(* Logix 5000 AddOnInstructionDefinition export Banner_Q90R_KD_Param_v4; software revision 33.00 *)

TYPE Banner_IOL_Port_v4 :   // UDT that has all of the data items necessary to communicate with a specific Port on a IO-Link Master
STRUCT
   Port_Controlled : INT;   // Each bit represents a port on an IO-Link Master. Set to 1 to tell AOI to control that port.
   Port_Activate : INT;   // Each bit represents a port on an IO-Link Master. When ON that port will process any commands in queue.
   Port_Read : INT;   // Each bit represents a port on an IO-Link Master. Used to determine when device AOI has requested a Read command.
   Port_Write : INT;   // Each bit represents a port on an IO-Link Master. Used to determine when device AOI has requested a Write command.
   Port_RW_Complete : INT;   // Each bit represents a port on an IO-Link Master. Tells device AOI that Read or Write request has been completed.
   Port_Device_Read : INT;
   Data_Transfer : SINT[190];   // Array to transfer data from IO-Master to device AOIs.
END_STRUCT
END_TYPE

TYPE Banner_Q90RKD_BDC_v4 :
STRUCT
   Setpoint_1 : DINT;   // 0 to 15000. SP1 switch point in Switch or Window mode.
   Setpoint_2 : DINT;   // 0 to 15000. SP2 switch point in Window mode only.
   Switchpoint : INT;   // 0 = Light Operate, 1 = Dark Operate
   Mode : SINT;   // 1 = Switch Mode/Single Mode, 2 = Window Mode
   Hysteresis : INT;   // 0 to 15000
   Delay_On : DINT;   // 0 to 60000 ms.
   Delay_Off : DINT;   // 0 to 60000 ms.
   Teach_Offset : DINT;   // -15000 to 15000. Offset applied to taught switch point during single point teach.
END_STRUCT
END_TYPE

TYPE Banner_Q90RKD_Config_v4 :
STRUCT
   Response_Speed : SINT;   // 0 = Fast, 1 = Medium, 2 = Slow
   Peak_Select_Mode : SINT;   // 0 = Strongest Peak, 1 = First Peak
   Output_Polarity : SINT;   // 0 = NPN, 1 = PNP
   Process_Data_Filter_Time : INT;   // Time in ms to average process data between updates.
   Process_Data_Layout : SINT;   // 0 = Digital Measurement Sensor, 1 = Distance and Excess Gain, 2 = Distance and Excess Gain with Binary
   Remote_Input_Mode : SINT;   // 0 = Disabled, 1 = Teach
   LEDs_Disabled : SINT;   // Q90R Only. 0 = Enabled, 1= Disabled.
   Amplitude_Threshold : DINT;   // 100 to 5000 for T30R and 100 to 10000 for Q90R.
   Limit_Filter_Enabled : SINT;   // 0 = Disabled, 1 = Enabled. Rate of change filter for the distance meansurement.
   Limit_Filter_Positive_Hold_Time : DINT;   // 50 to 3600000. Hold time for when distance change exceeds positive window.
   Limit_Filter_Negative_Hold_Time : DINT;   // 50 to 3600000. Hold time for when distance change exceeds negative window.
   Limit_Filter_Positive_Distance : DINT;   // 0 to 1000. Window size for distance changes going away from sensor (set 0 to disable)
   Limit_Filter_Negative_Distance : DINT;   // 0 to 1000. Window size for distance changes going towards sensor (set 0 to disable)
   Secondary_Output_Mode : SINT;   // 0 = Independent Output, 1 = Complementary Output, 2 = Pulse Frequency Output
END_STRUCT
END_TYPE

TYPE Banner_Q90RKD_Direct_v4 :
STRUCT
   Master_Cycle_Time : INT;
   Min_Cycle_Time : INT;
   M_Sequence_Capability : INT;
   IO_Link_Version_ID : INT;
   Process_Data_Input_Length : INT;
   Process_Data_Output_Length : INT;
   Combined_Vendor_ID : DINT;   // IO-Link Vendor ID
   Vendor_ID1 : INT;
   Vendor_ID2 : INT;
   Combined_Device_ID : DINT;   // IO-Link Device ID
   Device_ID1 : INT;
   Device_ID2 : INT;
   Device_ID3 : INT;
END_STRUCT
END_TYPE

TYPE Banner_Q90RKD_RD_v4 :   // UDT that stores the Read Data for a Q90RKD.
STRUCT
   Direct : Banner_Q90RKD_Direct_v4;
   Serial_Number : STRING;
   Teach_State : SINT;   // 0 = Idle, 1 = SP1 Success, 2 = SP2 Success, 3 = SP1 SP2 Success, 4 = Wait for command, 5 = Busy, 7 = Error
   SP1_TP1 : SINT;
   SP1_TP2 : SINT;
   SP2_TP1 : SINT;
   SP2_TP2 : SINT;
   Status : Banner_Q90RKD_Status_v4;
   All_Time_Run_Time : DINT;   // Read only counter that tracks the total time sensor has been running since manufacture. Value in Hours.
   MDC_Lower_Limit : DINT;
   MDC_Upper_Limit : DINT;
   MDC_Unit : INT;
   MDC_Scale : SINT;
END_STRUCT
END_TYPE

TYPE Banner_Q90RKD_Status_v4 :
STRUCT
   Distance_Meaurement : DINT;
   Excess_Gain : DINT;   // Amount of singal measured over the minimum threshold.
   Stability : SINT;   // 0 = No target, 1 = Marginal target, 2 = Strong target.
   Fault_Status : SINT;   // 0 = No Fault, 1 = Fault Present
   Temperature : DINT;   // Internal Temperature.
   Last_Taught_Temperature : DINT;   // Internal Temperature the last time device was taught.
END_STRUCT
END_TYPE

TYPE Banner_Q90RKD_v4 :   // All of the parameters for a Q90RKD.
STRUCT
   Initial_Global_Read : BOOL;   // Determines if all of the IO-Link data has been read into the PLC yet
   Command : INT;   // Value placed in here will activate a read or write to a specifc IO-Link Index
   Read : Banner_Q90RKD_RD_v4;   // Read Only Data
   Write : Banner_Q90RKD_WD_v4;   // Write Data
   Archive : Banner_Q90RKD_WD_v4;   // Archive Data
   Reset : BOOL;   // Resets AOI. This will force a complete parameter read of the sensor.
END_STRUCT
END_TYPE

TYPE Banner_Q90RKD_WD_v4 :   // UDT that stores the Write Data for a Q90RKD.
STRUCT
   System_Command : INT;   // See IODD file for list of commands that can be activated via the System Command interface
   Teach_in_Channel : SINT;   // 0 = Default, 1 = BDC1, 2 = BDC2
   BDC1 : Banner_Q90RKD_BDC_v4;
   BDC2 : Banner_Q90RKD_BDC_v4;
   Config : Banner_Q90RKD_Config_v4;
   Resettable_Run_Time : DINT;
   Loss_of_Signal : SINT;   // 0 = Hold, 1 = Low, 2 = High
   SP1_PFM_Setpoint : DINT;   // 0 to 15000 in Hz
   SP2_PFM_Setpoint : DINT;   // 0 to 15000 in Hz
   All_Time_Run_Time_Event_Time : DINT;
   Resettable_Run_Time_Event_Time : DINT;
   Active_Sensing_Range_Near : DINT;   // 0 to 16000. Near measurement limit of sensing range.
   Active_Sensing_Range_Far : DINT;   // 0 to 16000. Far measurement limit of sensing range.
END_STRUCT
END_TYPE

ADD_ON_INSTRUCTION Banner_Q90R_KD_Param_v4   (* revision 4.0, vendor Banner Engineering *)
// AOI to read and write parameter data to an IO-Link Q90R Dual Discrete.
VAR_IN_OUT
   Q90RKD : Banner_Q90RKD_v4; {required}
   Port_Data : Banner_IOL_Port_v4; {required}
END_VAR
VAR_INPUT
   Port : DINT; {required}
END_VAR
VAR
   Local_Control : DINT; {access None}
   Global_Read_Command_Value : INT; {access None}
   Global_Write_Command_Value : INT; {access None}
   Command_Being_Processed : BOOL; {access None}
   Update_Archive : BOOL; {access None}
   Index_Write_Inprocess : DINT; {access None}
   Index_Write_Control : DINT; {access None}
   Inprocess_Index : DINT; {access None}
END_VAR

ROUTINE Logic   (* ladder *)
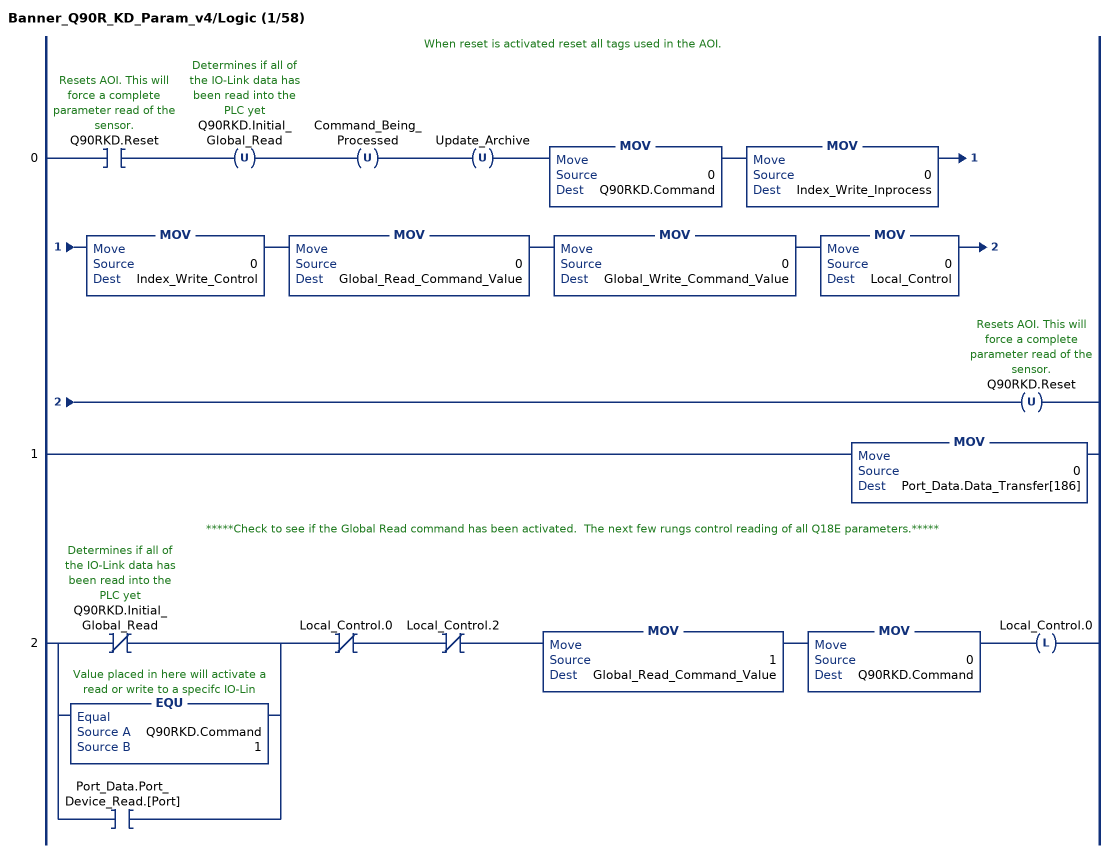
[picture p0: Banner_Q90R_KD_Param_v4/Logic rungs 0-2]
   // When reset is activated reset all tags used in the AOI.
   0: XIC(Q90RKD.Reset)OTU(Q90RKD.Initial_Global_Read)OTU(Command_Being_Processed)OTU(Update_Archive)MOV(0,Q90RKD.Command)MOV(0,Index_Write_Inprocess)MOV(0,Index_Write_Control)MOV(0,Global_Read_Command_Value)MOV(0,Global_Write_Command_Value)MOV(0,Local_Control)OTU(Q90RKD.Reset);
   1: MOV(0,Port_Data.Data_Transfer[186]);
   // *****Check to see if the Global Read command has been activated.  The next few rungs control reading of all Q18E parameters.*****
   2: [XIO(Q90RKD.Initial_Global_Read) ,EQU(Q90RKD.Command,1) ,XIC(Port_Data.Port_Device_Read.[Port]) ]XIO(Local_Control.0)XIO(Local_Control.2)MOV(1,Global_Read_Command_Value)MOV(0,Q90RKD.Command)OTL(Local_Control.0);
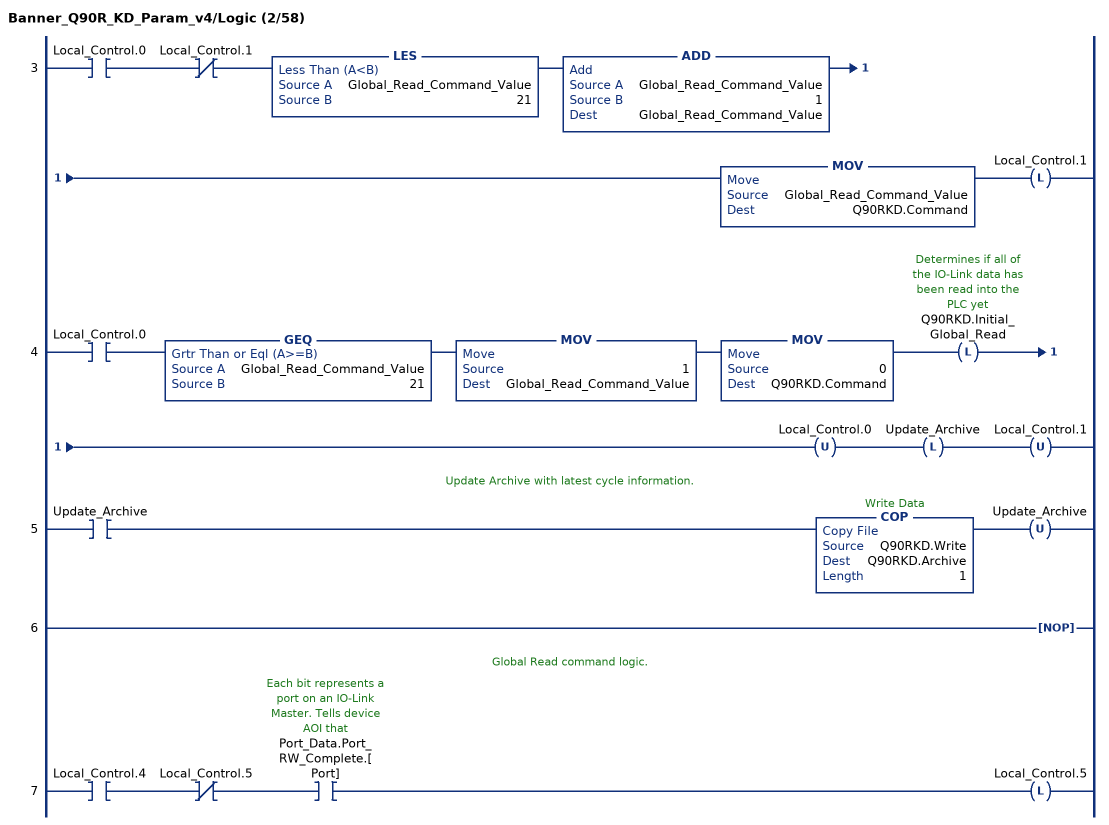
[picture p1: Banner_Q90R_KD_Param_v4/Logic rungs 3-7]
   3: XIC(Local_Control.0)XIO(Local_Control.1)LES(Global_Read_Command_Value,21)ADD(Global_Read_Command_Value,1,Global_Read_Command_Value)MOV(Global_Read_Command_Value,Q90RKD.Command)OTL(Local_Control.1);
   4: XIC(Local_Control.0)GEQ(Global_Read_Command_Value,21)MOV(1,Global_Read_Command_Value)MOV(0,Q90RKD.Command)OTL(Q90RKD.Initial_Global_Read)OTU(Local_Control.0)OTL(Update_Archive)OTU(Local_Control.1);
   // Update Archive with latest cycle information.
   5: XIC(Update_Archive)COP(Q90RKD.Write,Q90RKD.Archive,1)OTU(Update_Archive);
   6: NOP();
   // Global Read command logic.
   7: XIC(Local_Control.4)XIO(Local_Control.5)XIC(Port_Data.Port_RW_Complete.[Port])OTL(Local_Control.5);
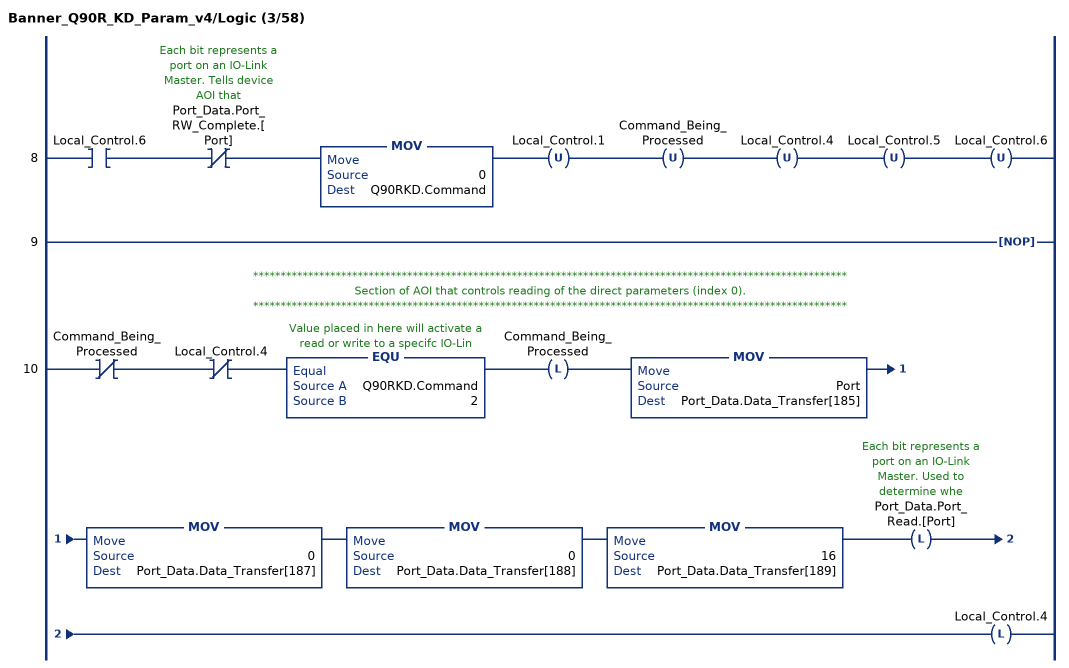
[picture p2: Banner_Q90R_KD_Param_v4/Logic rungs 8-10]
   8: XIC(Local_Control.6)XIO(Port_Data.Port_RW_Complete.[Port])MOV(0,Q90RKD.Command)OTU(Local_Control.1)OTU(Command_Being_Processed)OTU(Local_Control.4)OTU(Local_Control.5)OTU(Local_Control.6);
   9: NOP();
   // ************************************************************************************************************
   // Section of AOI that controls reading of the direct parameters (index 0).
   // ************************************************************************************************************
   10: XIO(Command_Being_Processed)XIO(Local_Control.4)EQU(Q90RKD.Command,2)OTL(Command_Being_Processed)MOV(Port,Port_Data.Data_Transfer[185])MOV(0,Port_Data.Data_Transfer[187])MOV(0,Port_Data.Data_Transfer[188])MOV(16,Port_Data.Data_Transfer[189])OTL(Port_Data.Port_Read.[Port])OTL(Local_Control.4);
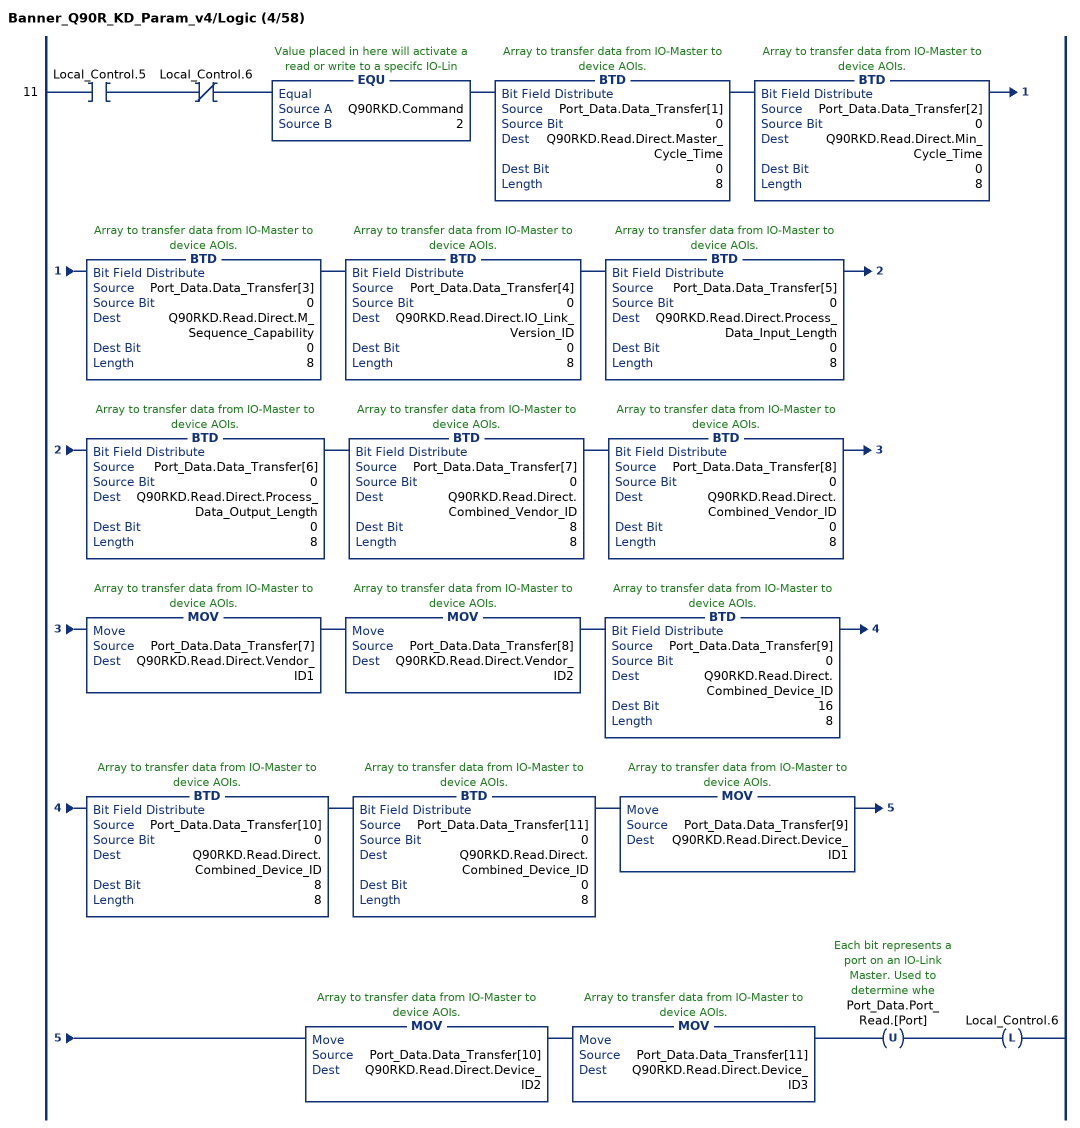
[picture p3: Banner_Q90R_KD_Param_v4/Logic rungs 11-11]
   11: XIC(Local_Control.5)XIO(Local_Control.6)EQU(Q90RKD.Command,2)BTD(Port_Data.Data_Transfer[1],0,Q90RKD.Read.Direct.Master_Cycle_Time,0,8)BTD(Port_Data.Data_Transfer[2],0,Q90RKD.Read.Direct.Min_Cycle_Time,0,8)BTD(Port_Data.Data_Transfer[3],0,Q90RKD.Read.Direct.M_Sequence_Capability,0,8)BTD(Port_Data.Data_Transfer[4],0,Q90RKD.Read.Direct.IO_Link_Version_ID,0,8)BTD(Port_Data.Data_Transfer[5],0,Q90RKD.Read.Direct.Process_Data_Input_Length,0,8)BTD(Port_Data.Data_Transfer[6],0,Q90RKD.Read.Direct.Process_Data_Output_Length,0,8)BTD(Port_Data.Data_Transfer[7],0,Q90RKD.Read.Direct.Combined_Vendor_ID,8,8)BTD(Port_Data.Data_Transfer[8],0,Q90RKD.Read.Direct.Combined_Vendor_ID,0,8)MOV(Port_Data.Data_Transfer[7],Q90RKD.Read.Direct.Vendor_ID1)MOV(Port_Data.Data_Transfer[8],Q90RKD.Read.Direct.Vendor_ID2)BTD(Port_Data.Data_Transfer[9],0,Q90RKD.Read.Direct.Combined_Device_ID,16,8)BTD(Port_Data.Data_Transfer[10],0,Q90RKD.Read.Direct.Combined_Device_ID,8,8)BTD(Port_Data.Data_Transfer[11],0,Q90RKD.Read.Direct.Combined_Device_ID,0,8)MOV(Port_Data.Data_Transfer[9],Q90RKD.Read.Direct.Device_ID1)MOV(Port_Data.Data_Transfer[10],Q90RKD.Read.Direct.Device_ID2)MOV(Port_Data.Data_Transfer[11],Q90RKD.Read.Direct.Device_ID3)OTU(Port_Data.Port_Read.[Port])OTL(Local_Control.6);
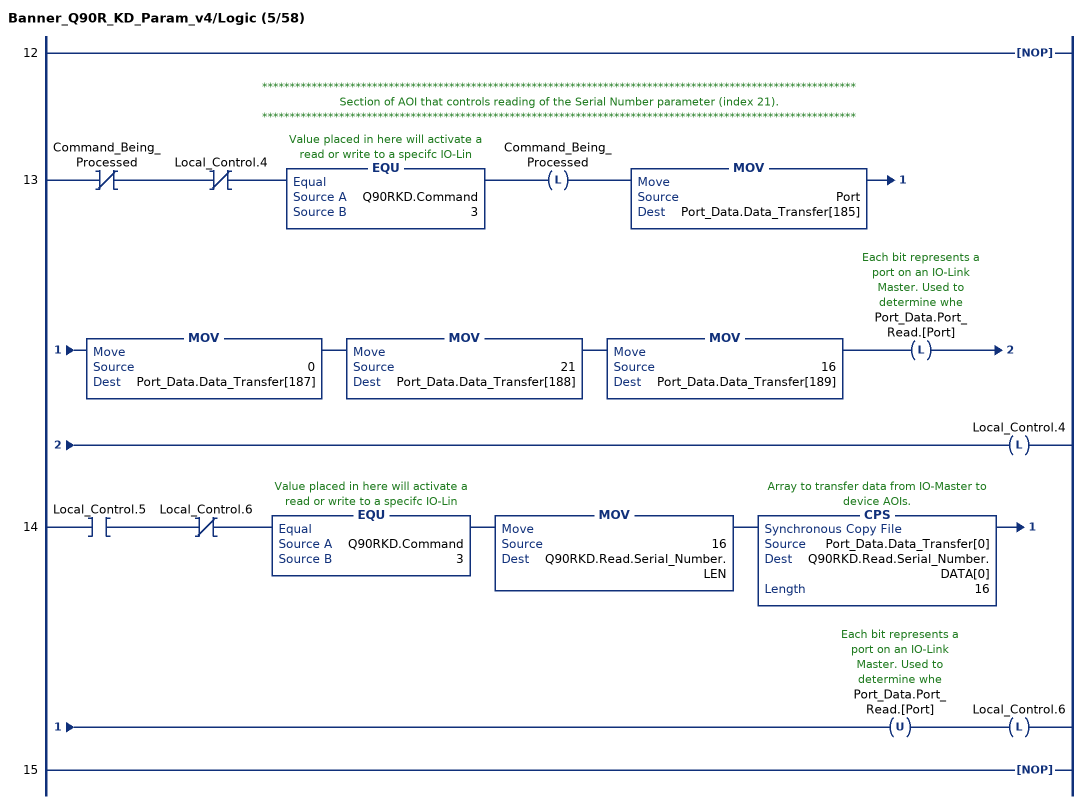
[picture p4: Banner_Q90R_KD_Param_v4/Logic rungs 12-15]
   12: NOP();
   // ************************************************************************************************************
   // Section of AOI that controls reading of the Serial Number parameter (index 21).
   // ************************************************************************************************************
   13: XIO(Command_Being_Processed)XIO(Local_Control.4)EQU(Q90RKD.Command,3)OTL(Command_Being_Processed)MOV(Port,Port_Data.Data_Transfer[185])MOV(0,Port_Data.Data_Transfer[187])MOV(21,Port_Data.Data_Transfer[188])MOV(16,Port_Data.Data_Transfer[189])OTL(Port_Data.Port_Read.[Port])OTL(Local_Control.4);
   14: XIC(Local_Control.5)XIO(Local_Control.6)EQU(Q90RKD.Command,3)MOV(16,Q90RKD.Read.Serial_Number.LEN)CPS(Port_Data.Data_Transfer[0],Q90RKD.Read.Serial_Number.DATA[0],16)OTU(Port_Data.Port_Read.[Port])OTL(Local_Control.6);
   15: NOP();
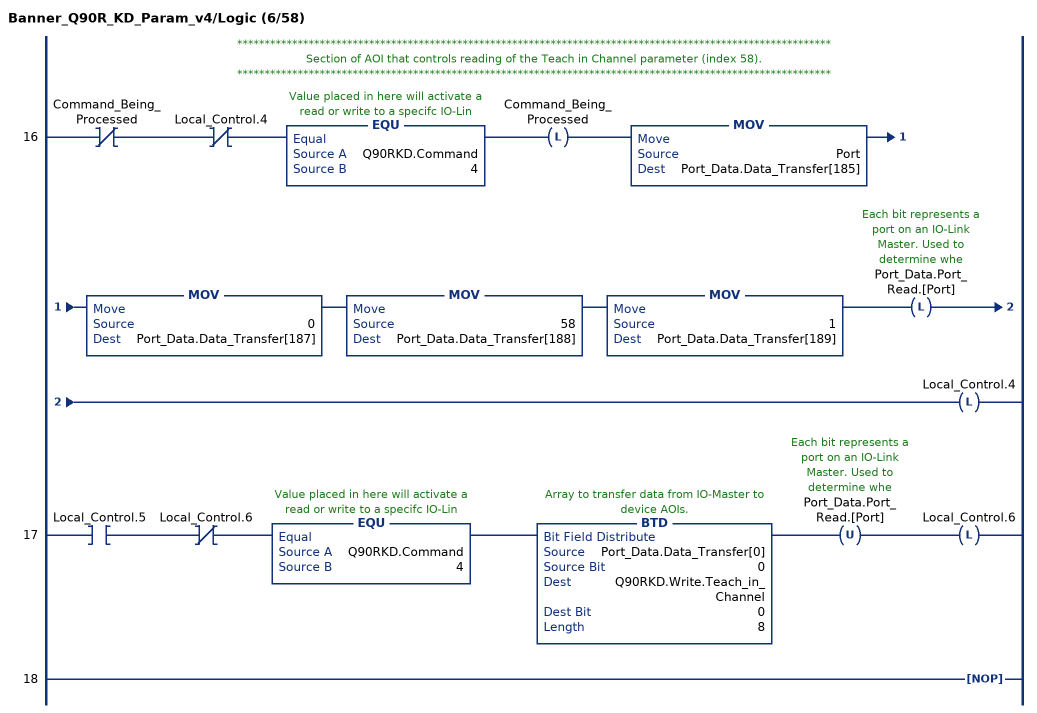
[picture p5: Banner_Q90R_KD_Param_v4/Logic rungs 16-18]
   // ************************************************************************************************************
   // Section of AOI that controls reading of the Teach in Channel parameter (index 58).
   // ************************************************************************************************************
   16: XIO(Command_Being_Processed)XIO(Local_Control.4)EQU(Q90RKD.Command,4)OTL(Command_Being_Processed)MOV(Port,Port_Data.Data_Transfer[185])MOV(0,Port_Data.Data_Transfer[187])MOV(58,Port_Data.Data_Transfer[188])MOV(1,Port_Data.Data_Transfer[189])OTL(Port_Data.Port_Read.[Port])OTL(Local_Control.4);
   17: XIC(Local_Control.5)XIO(Local_Control.6)EQU(Q90RKD.Command,4)BTD(Port_Data.Data_Transfer[0],0,Q90RKD.Write.Teach_in_Channel,0,8)OTU(Port_Data.Port_Read.[Port])OTL(Local_Control.6);
   18: NOP();
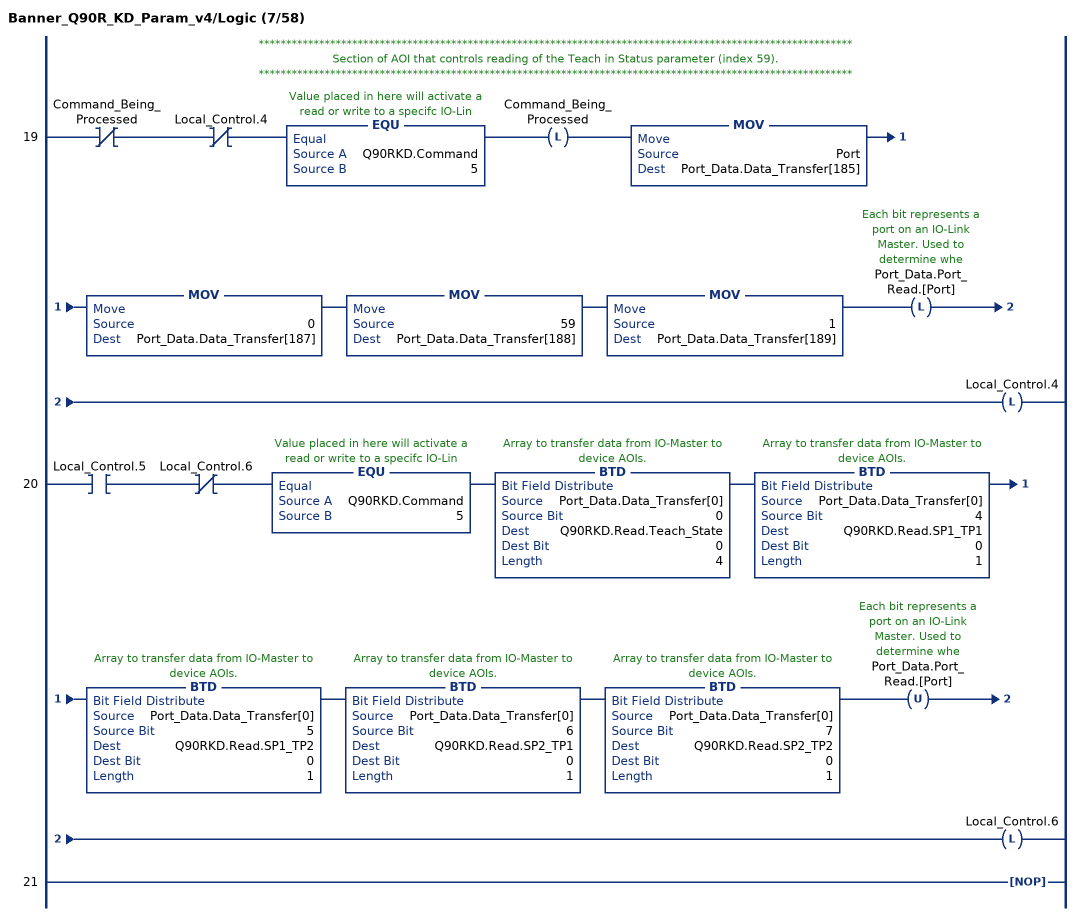
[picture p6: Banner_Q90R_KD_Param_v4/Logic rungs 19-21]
   // ************************************************************************************************************
   // Section of AOI that controls reading of the Teach in Status parameter (index 59).
   // ************************************************************************************************************
   19: XIO(Command_Being_Processed)XIO(Local_Control.4)EQU(Q90RKD.Command,5)OTL(Command_Being_Processed)MOV(Port,Port_Data.Data_Transfer[185])MOV(0,Port_Data.Data_Transfer[187])MOV(59,Port_Data.Data_Transfer[188])MOV(1,Port_Data.Data_Transfer[189])OTL(Port_Data.Port_Read.[Port])OTL(Local_Control.4);
   20: XIC(Local_Control.5)XIO(Local_Control.6)EQU(Q90RKD.Command,5)BTD(Port_Data.Data_Transfer[0],0,Q90RKD.Read.Teach_State,0,4)BTD(Port_Data.Data_Transfer[0],4,Q90RKD.Read.SP1_TP1,0,1)BTD(Port_Data.Data_Transfer[0],5,Q90RKD.Read.SP1_TP2,0,1)BTD(Port_Data.Data_Transfer[0],6,Q90RKD.Read.SP2_TP1,0,1)BTD(Port_Data.Data_Transfer[0],7,Q90RKD.Read.SP2_TP2,0,1)OTU(Port_Data.Port_Read.[Port])OTL(Local_Control.6);
   21: NOP();
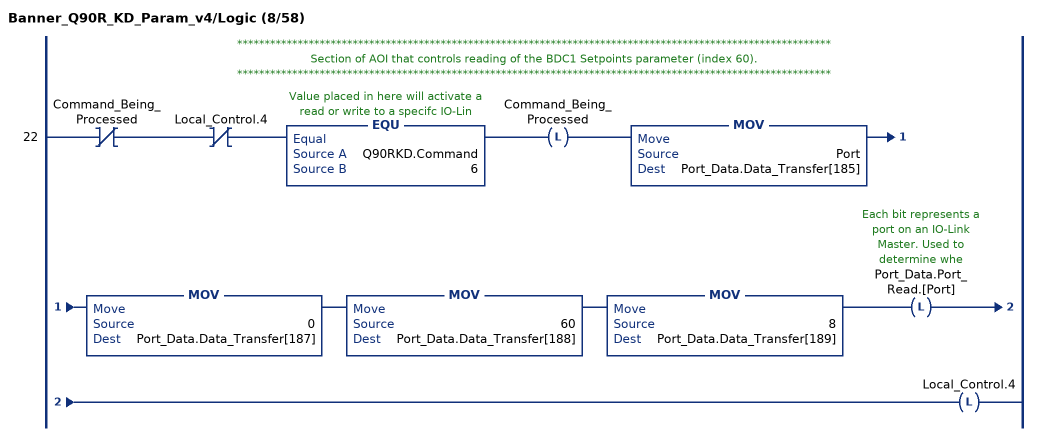
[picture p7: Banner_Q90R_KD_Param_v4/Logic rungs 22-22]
   // ************************************************************************************************************
   // Section of AOI that controls reading of the BDC1 Setpoints parameter (index 60).
   // ************************************************************************************************************
   22: XIO(Command_Being_Processed)XIO(Local_Control.4)EQU(Q90RKD.Command,6)OTL(Command_Being_Processed)MOV(Port,Port_Data.Data_Transfer[185])MOV(0,Port_Data.Data_Transfer[187])MOV(60,Port_Data.Data_Transfer[188])MOV(8,Port_Data.Data_Transfer[189])OTL(Port_Data.Port_Read.[Port])OTL(Local_Control.4);
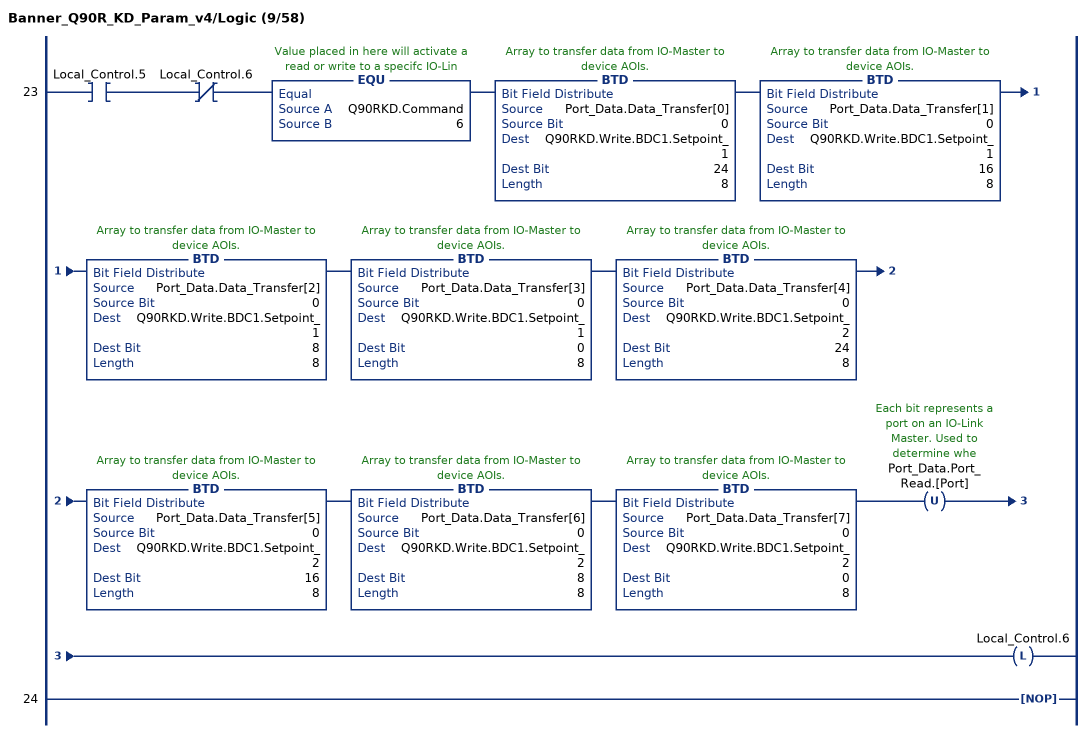
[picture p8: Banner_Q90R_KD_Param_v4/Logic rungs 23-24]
   23: XIC(Local_Control.5)XIO(Local_Control.6)EQU(Q90RKD.Command,6)BTD(Port_Data.Data_Transfer[0],0,Q90RKD.Write.BDC1.Setpoint_1,24,8)BTD(Port_Data.Data_Transfer[1],0,Q90RKD.Write.BDC1.Setpoint_1,16,8)BTD(Port_Data.Data_Transfer[2],0,Q90RKD.Write.BDC1.Setpoint_1,8,8)BTD(Port_Data.Data_Transfer[3],0,Q90RKD.Write.BDC1.Setpoint_1,0,8)BTD(Port_Data.Data_Transfer[4],0,Q90RKD.Write.BDC1.Setpoint_2,24,8)BTD(Port_Data.Data_Transfer[5],0,Q90RKD.Write.BDC1.Setpoint_2,16,8)BTD(Port_Data.Data_Transfer[6],0,Q90RKD.Write.BDC1.Setpoint_2,8,8)BTD(Port_Data.Data_Transfer[7],0,Q90RKD.Write.BDC1.Setpoint_2,0,8)OTU(Port_Data.Port_Read.[Port])OTL(Local_Control.6);
   24: NOP();
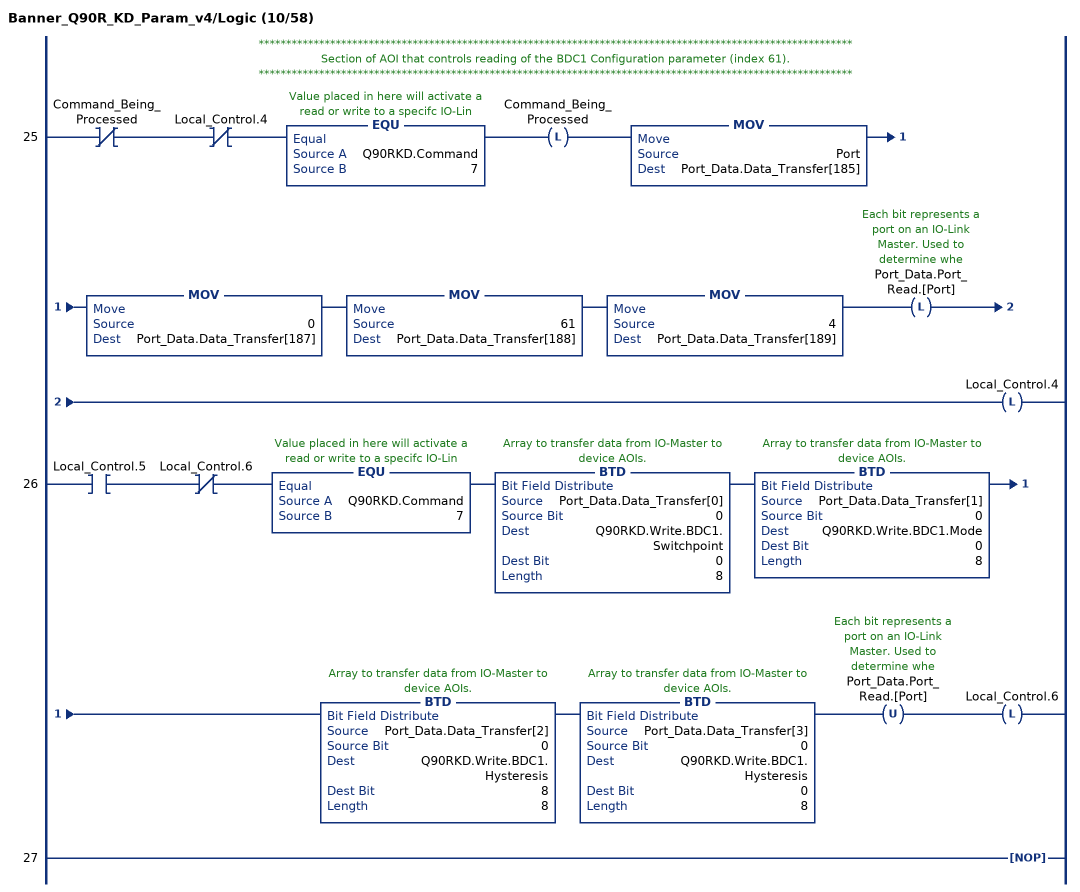
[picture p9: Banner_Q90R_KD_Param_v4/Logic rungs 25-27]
   // ************************************************************************************************************
   // Section of AOI that controls reading of the BDC1 Configuration parameter (index 61).
   // ************************************************************************************************************
   25: XIO(Command_Being_Processed)XIO(Local_Control.4)EQU(Q90RKD.Command,7)OTL(Command_Being_Processed)MOV(Port,Port_Data.Data_Transfer[185])MOV(0,Port_Data.Data_Transfer[187])MOV(61,Port_Data.Data_Transfer[188])MOV(4,Port_Data.Data_Transfer[189])OTL(Port_Data.Port_Read.[Port])OTL(Local_Control.4);
   26: XIC(Local_Control.5)XIO(Local_Control.6)EQU(Q90RKD.Command,7)BTD(Port_Data.Data_Transfer[0],0,Q90RKD.Write.BDC1.Switchpoint,0,8)BTD(Port_Data.Data_Transfer[1],0,Q90RKD.Write.BDC1.Mode,0,8)BTD(Port_Data.Data_Transfer[2],0,Q90RKD.Write.BDC1.Hysteresis,8,8)BTD(Port_Data.Data_Transfer[3],0,Q90RKD.Write.BDC1.Hysteresis,0,8)OTU(Port_Data.Port_Read.[Port])OTL(Local_Control.6);
   27: NOP();
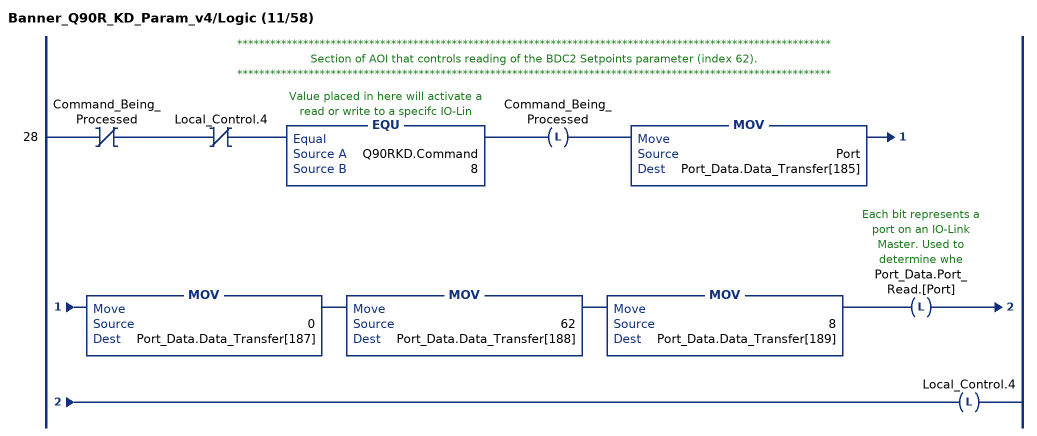
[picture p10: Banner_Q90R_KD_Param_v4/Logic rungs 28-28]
   // ************************************************************************************************************
   // Section of AOI that controls reading of the BDC2 Setpoints parameter (index 62).
   // ************************************************************************************************************
   28: XIO(Command_Being_Processed)XIO(Local_Control.4)EQU(Q90RKD.Command,8)OTL(Command_Being_Processed)MOV(Port,Port_Data.Data_Transfer[185])MOV(0,Port_Data.Data_Transfer[187])MOV(62,Port_Data.Data_Transfer[188])MOV(8,Port_Data.Data_Transfer[189])OTL(Port_Data.Port_Read.[Port])OTL(Local_Control.4);
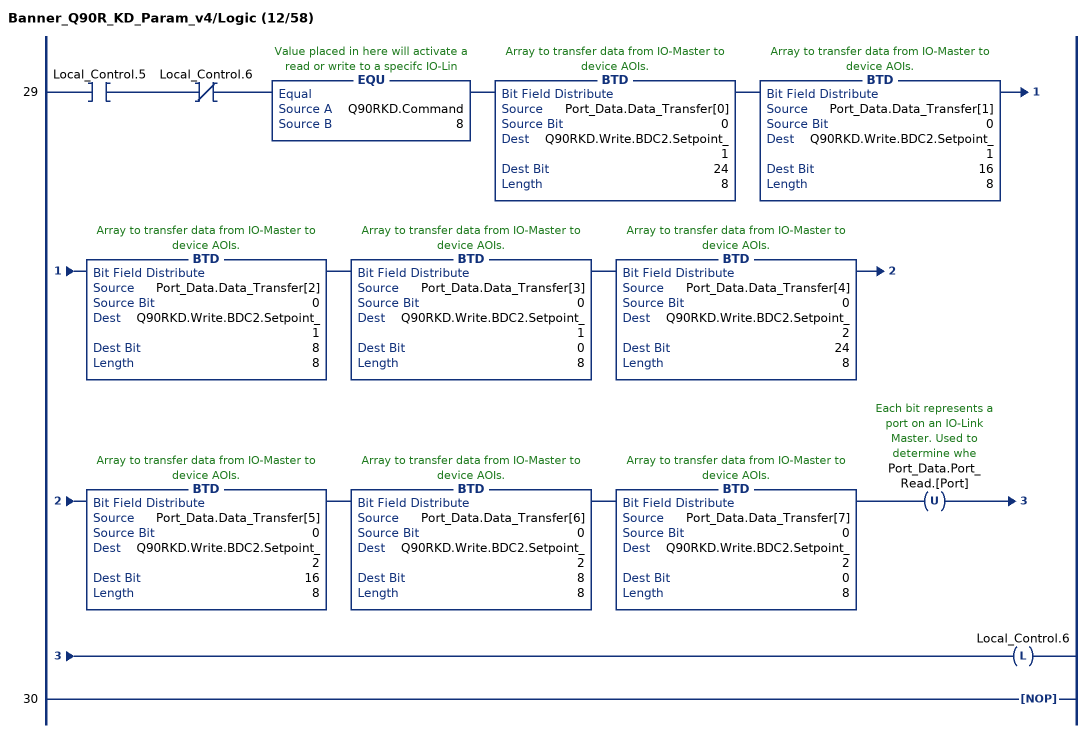
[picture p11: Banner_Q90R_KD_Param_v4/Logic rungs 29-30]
   29: XIC(Local_Control.5)XIO(Local_Control.6)EQU(Q90RKD.Command,8)BTD(Port_Data.Data_Transfer[0],0,Q90RKD.Write.BDC2.Setpoint_1,24,8)BTD(Port_Data.Data_Transfer[1],0,Q90RKD.Write.BDC2.Setpoint_1,16,8)BTD(Port_Data.Data_Transfer[2],0,Q90RKD.Write.BDC2.Setpoint_1,8,8)BTD(Port_Data.Data_Transfer[3],0,Q90RKD.Write.BDC2.Setpoint_1,0,8)BTD(Port_Data.Data_Transfer[4],0,Q90RKD.Write.BDC2.Setpoint_2,24,8)BTD(Port_Data.Data_Transfer[5],0,Q90RKD.Write.BDC2.Setpoint_2,16,8)BTD(Port_Data.Data_Transfer[6],0,Q90RKD.Write.BDC2.Setpoint_2,8,8)BTD(Port_Data.Data_Transfer[7],0,Q90RKD.Write.BDC2.Setpoint_2,0,8)OTU(Port_Data.Port_Read.[Port])OTL(Local_Control.6);
   30: NOP();
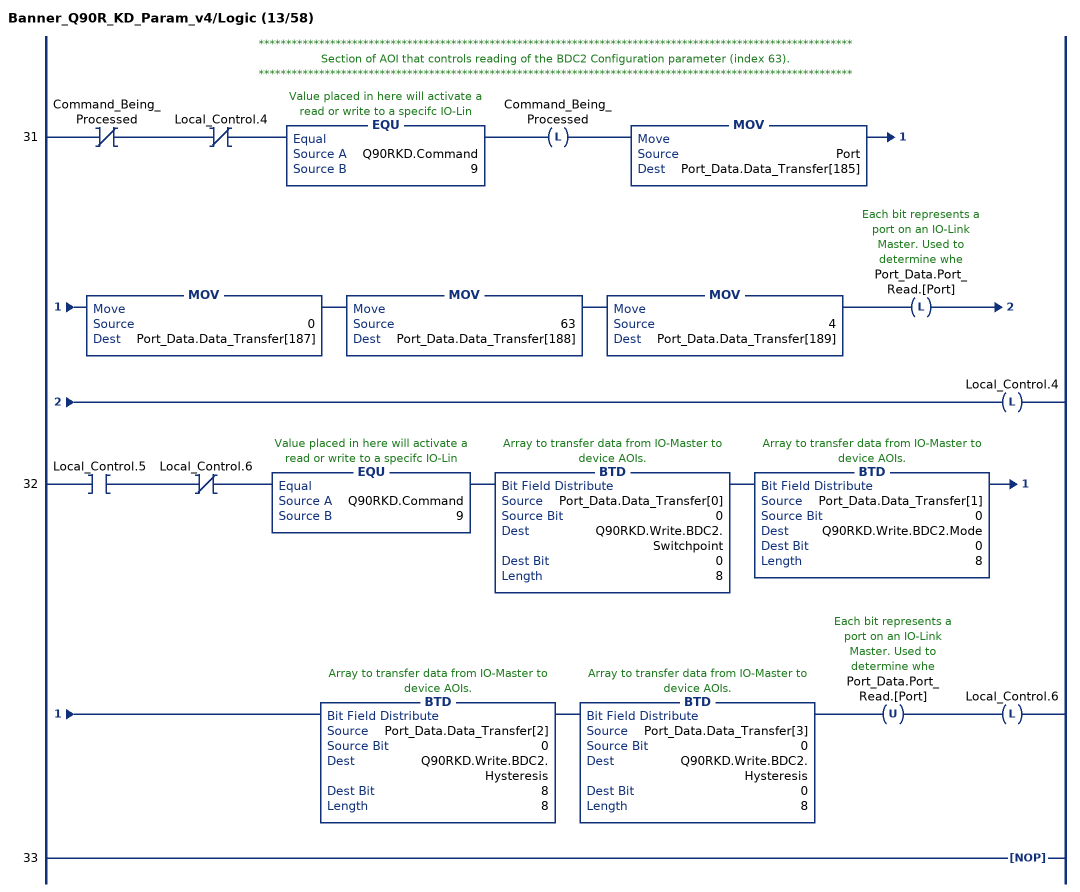
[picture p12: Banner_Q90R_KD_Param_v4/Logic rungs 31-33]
   // ************************************************************************************************************
   // Section of AOI that controls reading of the BDC2 Configuration parameter (index 63).
   // ************************************************************************************************************
   31: XIO(Command_Being_Processed)XIO(Local_Control.4)EQU(Q90RKD.Command,9)OTL(Command_Being_Processed)MOV(Port,Port_Data.Data_Transfer[185])MOV(0,Port_Data.Data_Transfer[187])MOV(63,Port_Data.Data_Transfer[188])MOV(4,Port_Data.Data_Transfer[189])OTL(Port_Data.Port_Read.[Port])OTL(Local_Control.4);
   32: XIC(Local_Control.5)XIO(Local_Control.6)EQU(Q90RKD.Command,9)BTD(Port_Data.Data_Transfer[0],0,Q90RKD.Write.BDC2.Switchpoint,0,8)BTD(Port_Data.Data_Transfer[1],0,Q90RKD.Write.BDC2.Mode,0,8)BTD(Port_Data.Data_Transfer[2],0,Q90RKD.Write.BDC2.Hysteresis,8,8)BTD(Port_Data.Data_Transfer[3],0,Q90RKD.Write.BDC2.Hysteresis,0,8)OTU(Port_Data.Port_Read.[Port])OTL(Local_Control.6);
   33: NOP();
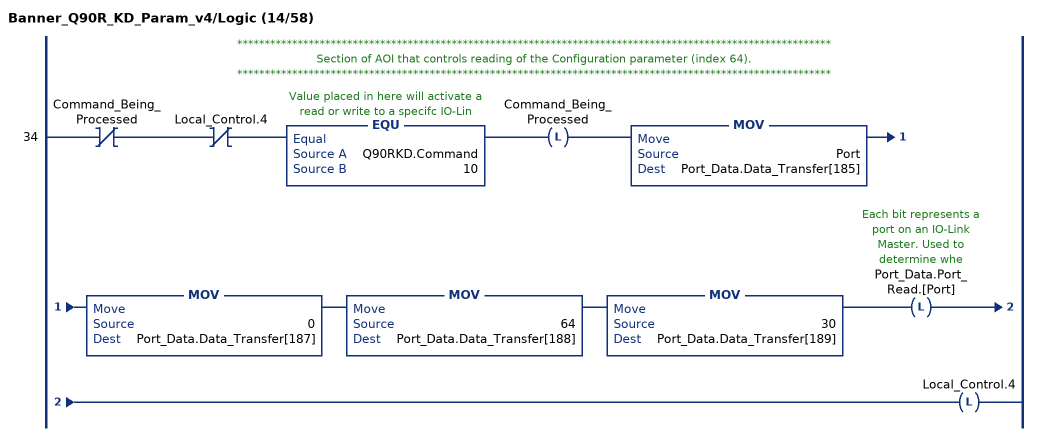
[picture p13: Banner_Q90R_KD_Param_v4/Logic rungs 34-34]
   // ************************************************************************************************************
   // Section of AOI that controls reading of the Configuration parameter (index 64).
   // ************************************************************************************************************
   34: XIO(Command_Being_Processed)XIO(Local_Control.4)EQU(Q90RKD.Command,10)OTL(Command_Being_Processed)MOV(Port,Port_Data.Data_Transfer[185])MOV(0,Port_Data.Data_Transfer[187])MOV(64,Port_Data.Data_Transfer[188])MOV(30,Port_Data.Data_Transfer[189])OTL(Port_Data.Port_Read.[Port])OTL(Local_Control.4);
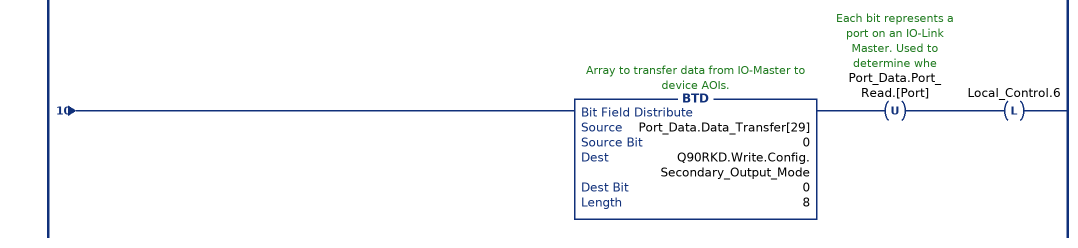
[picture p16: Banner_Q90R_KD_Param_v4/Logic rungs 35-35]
   35: XIC(Local_Control.5)XIO(Local_Control.6)EQU(Q90RKD.Command,10)BTD(Port_Data.Data_Transfer[0],0,Q90RKD.Write.Config.Response_Speed,0,8)BTD(Port_Data.Data_Transfer[1],0,Q90RKD.Write.Config.Peak_Select_Mode,0,8)BTD(Port_Data.Data_Transfer[2],0,Q90RKD.Write.Config.Output_Polarity,0,8)BTD(Port_Data.Data_Transfer[3],0,Q90RKD.Write.Config.Process_Data_Filter_Time,8,8)BTD(Port_Data.Data_Transfer[4],0,Q90RKD.Write.Config.Process_Data_Filter_Time,0,8)BTD(Port_Data.Data_Transfer[5],0,Q90RKD.Write.Config.Process_Data_Layout,0,8)BTD(Port_Data.Data_Transfer[6],0,Q90RKD.Write.Config.Remote_Input_Mode,0,8)BTD(Port_Data.Data_Transfer[7],0,Q90RKD.Write.Config.LEDs_Disabled,0,8)BTD(Port_Data.Data_Transfer[8],0,Q90RKD.Write.Config.Amplitude_Threshold,24,8)BTD(Port_Data.Data_Transfer[9],0,Q90RKD.Write.Config.Amplitude_Threshold,16,8)BTD(Port_Data.Data_Transfer[10],0,Q90RKD.Write.Config.Amplitude_Threshold,8,8)BTD(Port_Data.Data_Transfer[11],0,Q90RKD.Write.Config.Amplitude_Threshold,0,8)BTD(Port_Data.Data_Transfer[12],0,Q90RKD.Write.Config.Limit_Filter_Enabled,0,8)BTD(Port_Data.Data_Transfer[13],0,Q90RKD.Write.Config.Limit_Filter_Positive_Hold_Time,24,8)BTD(Port_Data.Data_Transfer[14],0,Q90RKD.Write.Config.Limit_Filter_Positive_Hold_Time,16,8)BTD(Port_Data.Data_Transfer[15],0,Q90RKD.Write.Config.Limit_Filter_Positive_Hold_Time,8,8)BTD(Port_Data.Data_Transfer[16],0,Q90RKD.Write.Config.Limit_Filter_Positive_Hold_Time,0,8)BTD(Port_Data.Data_Transfer[17],0,Q90RKD.Write.Config.Limit_Filter_Negative_Hold_Time,24,8)BTD(Port_Data.Data_Transfer[18],0,Q90RKD.Write.Config.Limit_Filter_Negative_Hold_Time,16,8)BTD(Port_Data.Data_Transfer[19],0,Q90RKD.Write.Config.Limit_Filter_Negative_Hold_Time,8,8)BTD(Port_Data.Data_Transfer[20],0,Q90RKD.Write.Config.Limit_Filter_Negative_Hold_Time,0,8)BTD(Port_Data.Data_Transfer[21],0,Q90RKD.Write.Config.Limit_Filter_Positive_Distance,24,8)BTD(Port_Data.Data_Transfer[22],0,Q90RKD.Write.Config.Limit_Filter_Positive_Distance,16,8)BTD(Port_Data.Data_Transfer[23],0,Q90RKD.Write.Config.Limit_Filter_Positive_Distance,8,8)BTD(Port_Data.Data_Transfer[24],0,Q90RKD.Write.Config.Limit_Filter_Positive_Distance,0,8)BTD(Port_Data.Data_Transfer[25],0,Q90RKD.Write.Config.Limit_Filter_Negative_Distance,24,8)BTD(Port_Data.Data_Transfer[26],0,Q90RKD.Write.Config.Limit_Filter_Negative_Distance,16,8)BTD(Port_Data.Data_Transfer[27],0,Q90RKD.Write.Config.Limit_Filter_Negative_Distance,8,8)BTD(Port_Data.Data_Transfer[28],0,Q90RKD.Write.Config.Limit_Filter_Negative_Distance,0,8)BTD(Port_Data.Data_Transfer[29],0,Q90RKD.Write.Config.Secondary_Output_Mode,0,8)OTU(Port_Data.Port_Read.[Port])OTL(Local_Control.6);
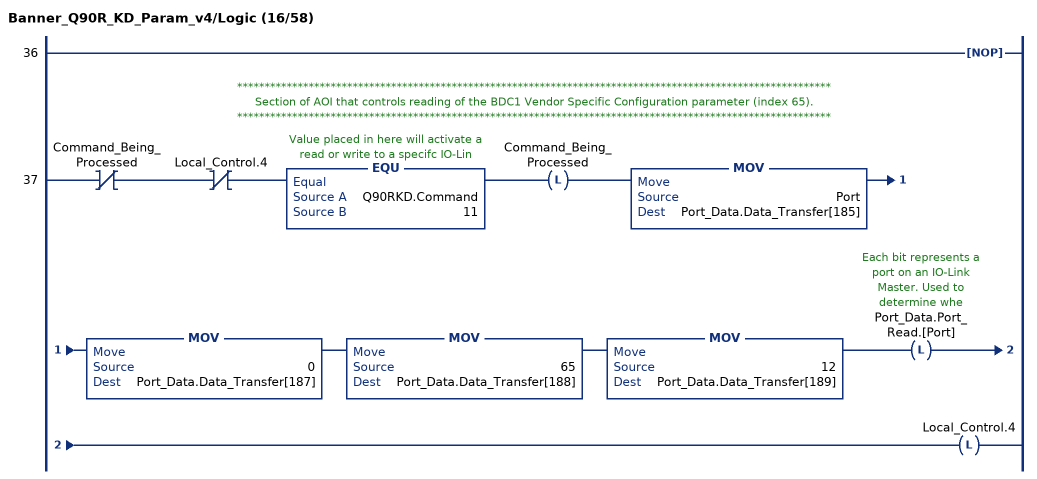
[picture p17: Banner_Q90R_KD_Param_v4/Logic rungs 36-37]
   36: NOP();
   // ************************************************************************************************************
   // Section of AOI that controls reading of the BDC1 Vendor Specific Configuration parameter (index 65).
   // ************************************************************************************************************
   37: XIO(Command_Being_Processed)XIO(Local_Control.4)EQU(Q90RKD.Command,11)OTL(Command_Being_Processed)MOV(Port,Port_Data.Data_Transfer[185])MOV(0,Port_Data.Data_Transfer[187])MOV(65,Port_Data.Data_Transfer[188])MOV(12,Port_Data.Data_Transfer[189])OTL(Port_Data.Port_Read.[Port])OTL(Local_Control.4);
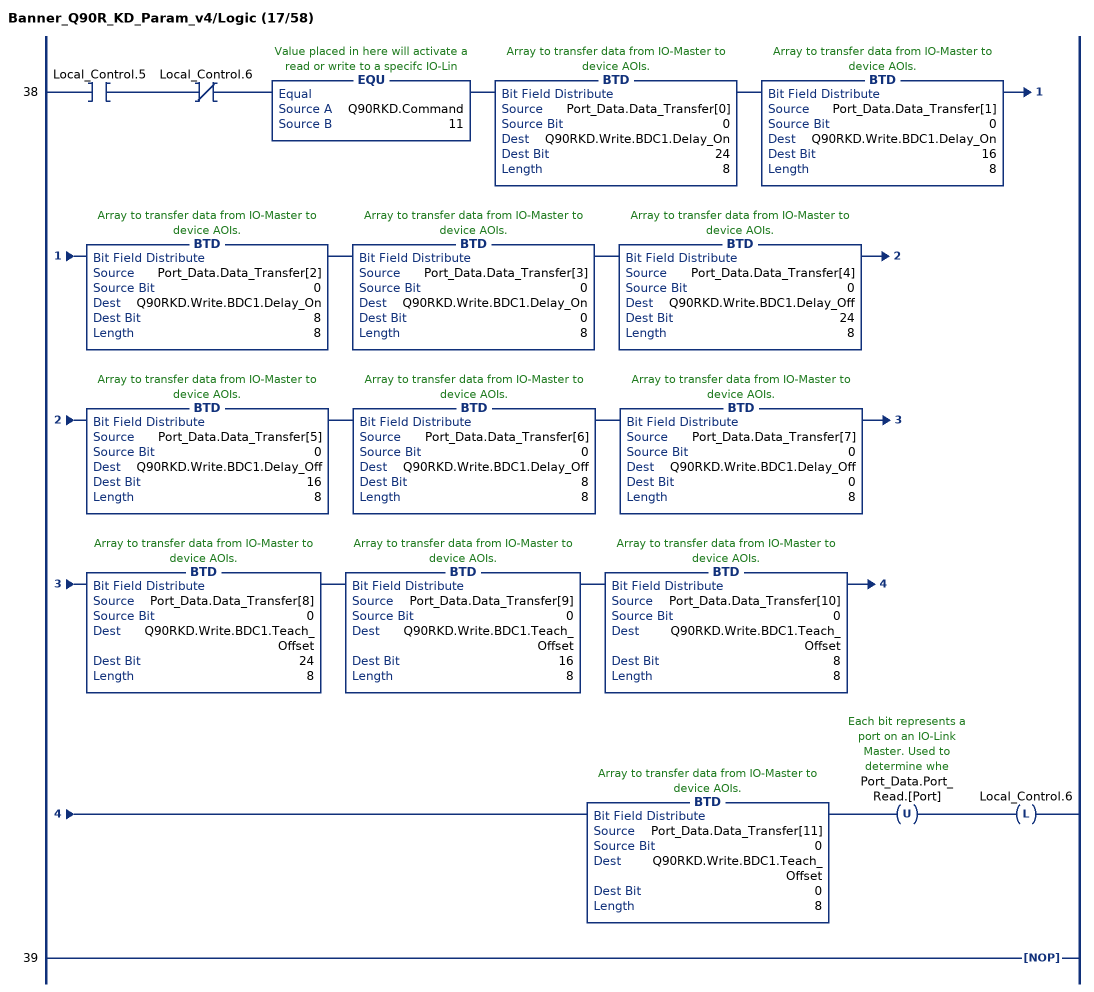
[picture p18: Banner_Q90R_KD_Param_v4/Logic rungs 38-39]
   38: XIC(Local_Control.5)XIO(Local_Control.6)EQU(Q90RKD.Command,11)BTD(Port_Data.Data_Transfer[0],0,Q90RKD.Write.BDC1.Delay_On,24,8)BTD(Port_Data.Data_Transfer[1],0,Q90RKD.Write.BDC1.Delay_On,16,8)BTD(Port_Data.Data_Transfer[2],0,Q90RKD.Write.BDC1.Delay_On,8,8)BTD(Port_Data.Data_Transfer[3],0,Q90RKD.Write.BDC1.Delay_On,0,8)BTD(Port_Data.Data_Transfer[4],0,Q90RKD.Write.BDC1.Delay_Off,24,8)BTD(Port_Data.Data_Transfer[5],0,Q90RKD.Write.BDC1.Delay_Off,16,8)BTD(Port_Data.Data_Transfer[6],0,Q90RKD.Write.BDC1.Delay_Off,8,8)BTD(Port_Data.Data_Transfer[7],0,Q90RKD.Write.BDC1.Delay_Off,0,8)BTD(Port_Data.Data_Transfer[8],0,Q90RKD.Write.BDC1.Teach_Offset,24,8)BTD(Port_Data.Data_Transfer[9],0,Q90RKD.Write.BDC1.Teach_Offset,16,8)BTD(Port_Data.Data_Transfer[10],0,Q90RKD.Write.BDC1.Teach_Offset,8,8)BTD(Port_Data.Data_Transfer[11],0,Q90RKD.Write.BDC1.Teach_Offset,0,8)OTU(Port_Data.Port_Read.[Port])OTL(Local_Control.6);
   39: NOP();
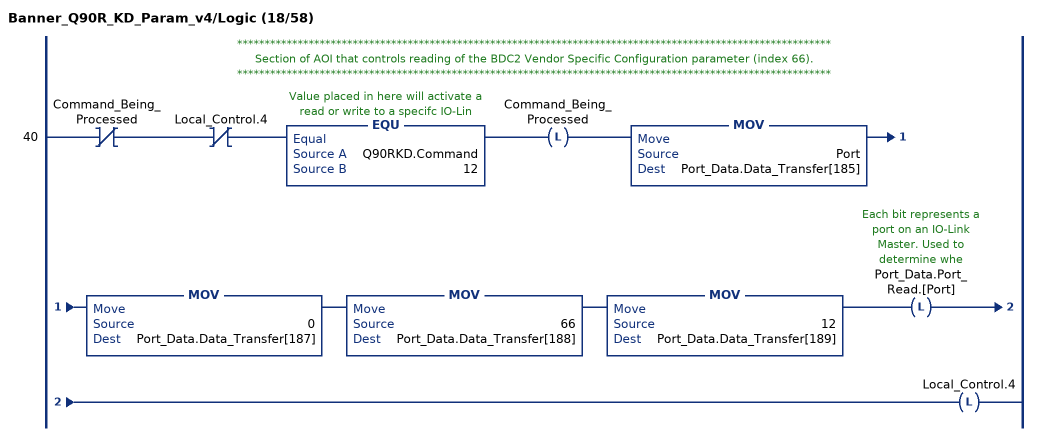
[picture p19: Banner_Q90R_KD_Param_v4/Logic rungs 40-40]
   // ************************************************************************************************************
   // Section of AOI that controls reading of the BDC2 Vendor Specific Configuration parameter (index 66).
   // ************************************************************************************************************
   40: XIO(Command_Being_Processed)XIO(Local_Control.4)EQU(Q90RKD.Command,12)OTL(Command_Being_Processed)MOV(Port,Port_Data.Data_Transfer[185])MOV(0,Port_Data.Data_Transfer[187])MOV(66,Port_Data.Data_Transfer[188])MOV(12,Port_Data.Data_Transfer[189])OTL(Port_Data.Port_Read.[Port])OTL(Local_Control.4);
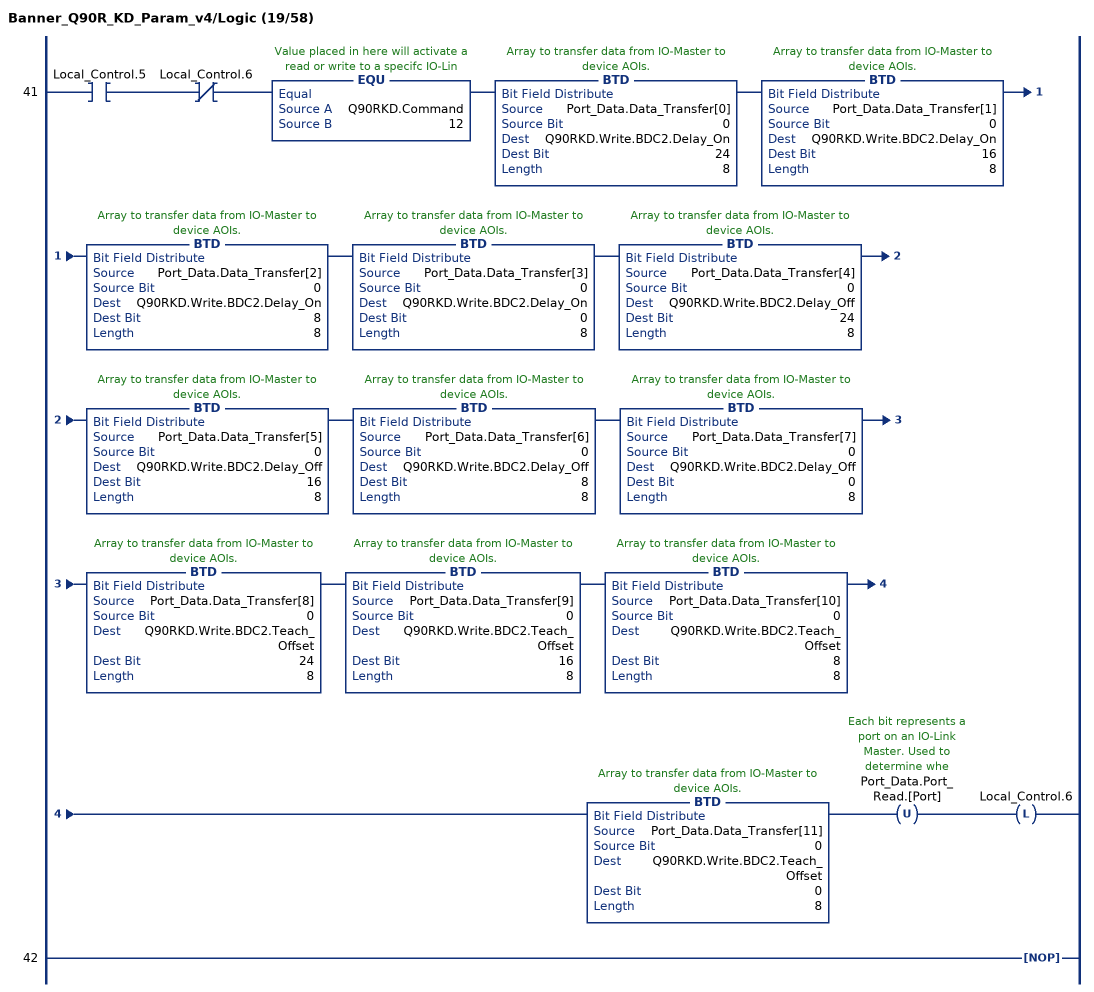
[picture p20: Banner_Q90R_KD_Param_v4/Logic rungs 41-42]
   41: XIC(Local_Control.5)XIO(Local_Control.6)EQU(Q90RKD.Command,12)BTD(Port_Data.Data_Transfer[0],0,Q90RKD.Write.BDC2.Delay_On,24,8)BTD(Port_Data.Data_Transfer[1],0,Q90RKD.Write.BDC2.Delay_On,16,8)BTD(Port_Data.Data_Transfer[2],0,Q90RKD.Write.BDC2.Delay_On,8,8)BTD(Port_Data.Data_Transfer[3],0,Q90RKD.Write.BDC2.Delay_On,0,8)BTD(Port_Data.Data_Transfer[4],0,Q90RKD.Write.BDC2.Delay_Off,24,8)BTD(Port_Data.Data_Transfer[5],0,Q90RKD.Write.BDC2.Delay_Off,16,8)BTD(Port_Data.Data_Transfer[6],0,Q90RKD.Write.BDC2.Delay_Off,8,8)BTD(Port_Data.Data_Transfer[7],0,Q90RKD.Write.BDC2.Delay_Off,0,8)BTD(Port_Data.Data_Transfer[8],0,Q90RKD.Write.BDC2.Teach_Offset,24,8)BTD(Port_Data.Data_Transfer[9],0,Q90RKD.Write.BDC2.Teach_Offset,16,8)BTD(Port_Data.Data_Transfer[10],0,Q90RKD.Write.BDC2.Teach_Offset,8,8)BTD(Port_Data.Data_Transfer[11],0,Q90RKD.Write.BDC2.Teach_Offset,0,8)OTU(Port_Data.Port_Read.[Port])OTL(Local_Control.6);
   42: NOP();
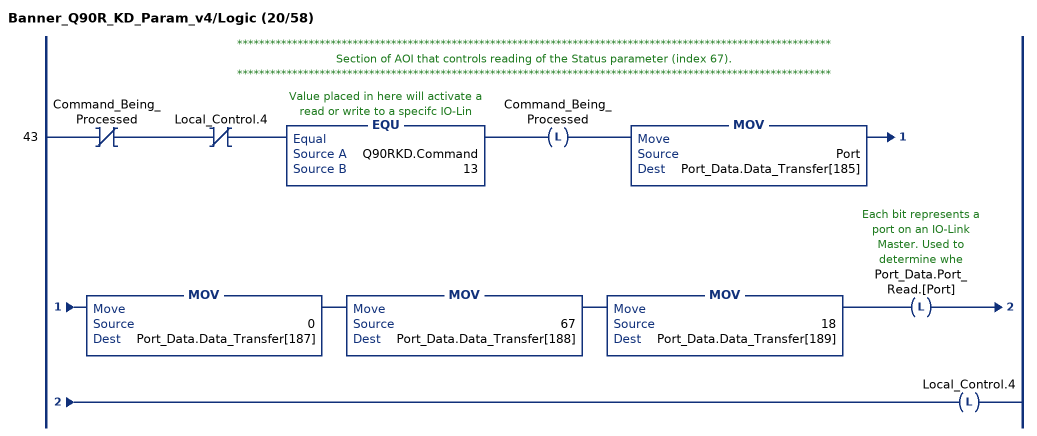
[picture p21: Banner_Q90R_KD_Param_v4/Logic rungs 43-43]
   // ************************************************************************************************************
   // Section of AOI that controls reading of the Status parameter (index 67).
   // ************************************************************************************************************
   43: XIO(Command_Being_Processed)XIO(Local_Control.4)EQU(Q90RKD.Command,13)OTL(Command_Being_Processed)MOV(Port,Port_Data.Data_Transfer[185])MOV(0,Port_Data.Data_Transfer[187])MOV(67,Port_Data.Data_Transfer[188])MOV(18,Port_Data.Data_Transfer[189])OTL(Port_Data.Port_Read.[Port])OTL(Local_Control.4);
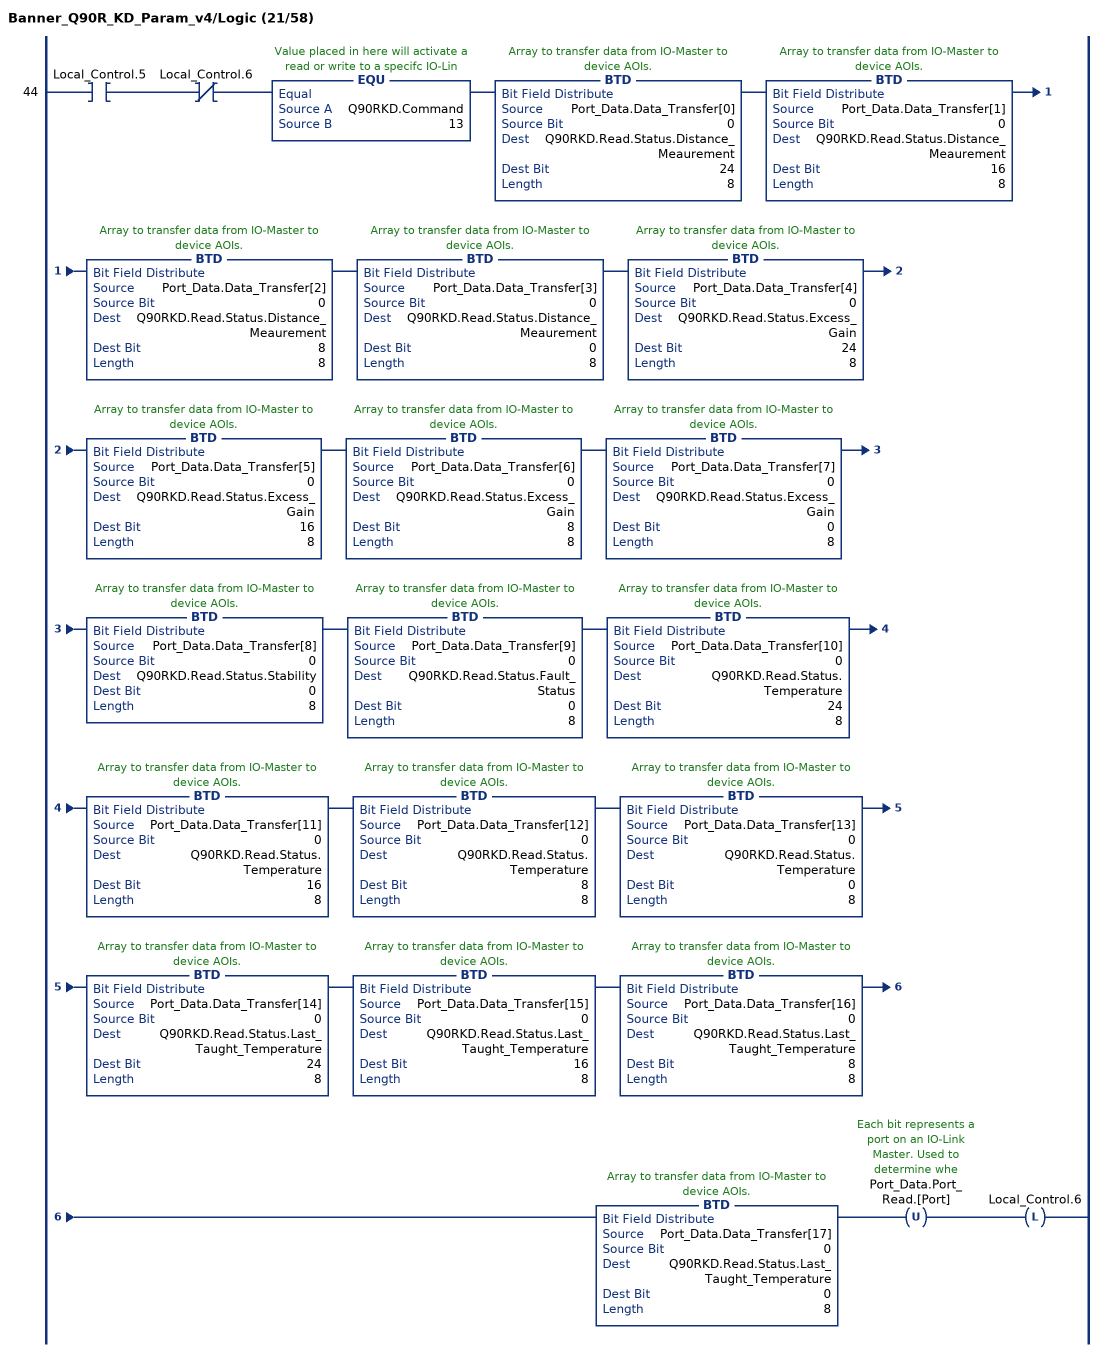
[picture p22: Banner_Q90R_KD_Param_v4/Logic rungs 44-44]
   44: XIC(Local_Control.5)XIO(Local_Control.6)EQU(Q90RKD.Command,13)BTD(Port_Data.Data_Transfer[0],0,Q90RKD.Read.Status.Distance_Meaurement,24,8)BTD(Port_Data.Data_Transfer[1],0,Q90RKD.Read.Status.Distance_Meaurement,16,8)BTD(Port_Data.Data_Transfer[2],0,Q90RKD.Read.Status.Distance_Meaurement,8,8)BTD(Port_Data.Data_Transfer[3],0,Q90RKD.Read.Status.Distance_Meaurement,0,8)BTD(Port_Data.Data_Transfer[4],0,Q90RKD.Read.Status.Excess_Gain,24,8)BTD(Port_Data.Data_Transfer[5],0,Q90RKD.Read.Status.Excess_Gain,16,8)BTD(Port_Data.Data_Transfer[6],0,Q90RKD.Read.Status.Excess_Gain,8,8)BTD(Port_Data.Data_Transfer[7],0,Q90RKD.Read.Status.Excess_Gain,0,8)BTD(Port_Data.Data_Transfer[8],0,Q90RKD.Read.Status.Stability,0,8)BTD(Port_Data.Data_Transfer[9],0,Q90RKD.Read.Status.Fault_Status,0,8)BTD(Port_Data.Data_Transfer[10],0,Q90RKD.Read.Status.Temperature,24,8)BTD(Port_Data.Data_Transfer[11],0,Q90RKD.Read.Status.Temperature,16,8)BTD(Port_Data.Data_Transfer[12],0,Q90RKD.Read.Status.Temperature,8,8)BTD(Port_Data.Data_Transfer[13],0,Q90RKD.Read.Status.Temperature,0,8)BTD(Port_Data.Data_Transfer[14],0,Q90RKD.Read.Status.Last_Taught_Temperature,24,8)BTD(Port_Data.Data_Transfer[15],0,Q90RKD.Read.Status.Last_Taught_Temperature,16,8)BTD(Port_Data.Data_Transfer[16],0,Q90RKD.Read.Status.Last_Taught_Temperature,8,8)BTD(Port_Data.Data_Transfer[17],0,Q90RKD.Read.Status.Last_Taught_Temperature,0,8)OTU(Port_Data.Port_Read.[Port])OTL(Local_Control.6);
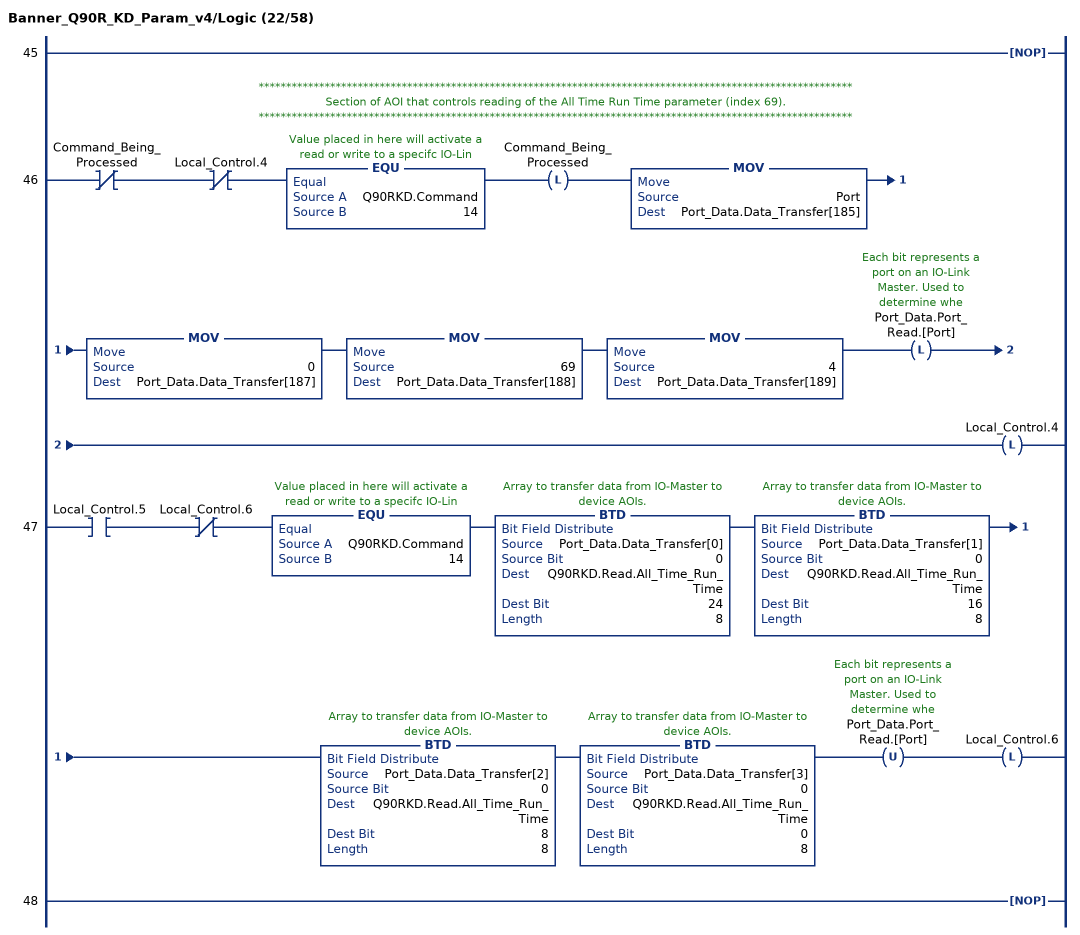
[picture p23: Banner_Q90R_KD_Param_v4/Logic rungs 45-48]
   45: NOP();
   // ************************************************************************************************************
   // Section of AOI that controls reading of the All Time Run Time parameter (index 69).
   // ************************************************************************************************************
   46: XIO(Command_Being_Processed)XIO(Local_Control.4)EQU(Q90RKD.Command,14)OTL(Command_Being_Processed)MOV(Port,Port_Data.Data_Transfer[185])MOV(0,Port_Data.Data_Transfer[187])MOV(69,Port_Data.Data_Transfer[188])MOV(4,Port_Data.Data_Transfer[189])OTL(Port_Data.Port_Read.[Port])OTL(Local_Control.4);
   47: XIC(Local_Control.5)XIO(Local_Control.6)EQU(Q90RKD.Command,14)BTD(Port_Data.Data_Transfer[0],0,Q90RKD.Read.All_Time_Run_Time,24,8)BTD(Port_Data.Data_Transfer[1],0,Q90RKD.Read.All_Time_Run_Time,16,8)BTD(Port_Data.Data_Transfer[2],0,Q90RKD.Read.All_Time_Run_Time,8,8)BTD(Port_Data.Data_Transfer[3],0,Q90RKD.Read.All_Time_Run_Time,0,8)OTU(Port_Data.Port_Read.[Port])OTL(Local_Control.6);
   48: NOP();
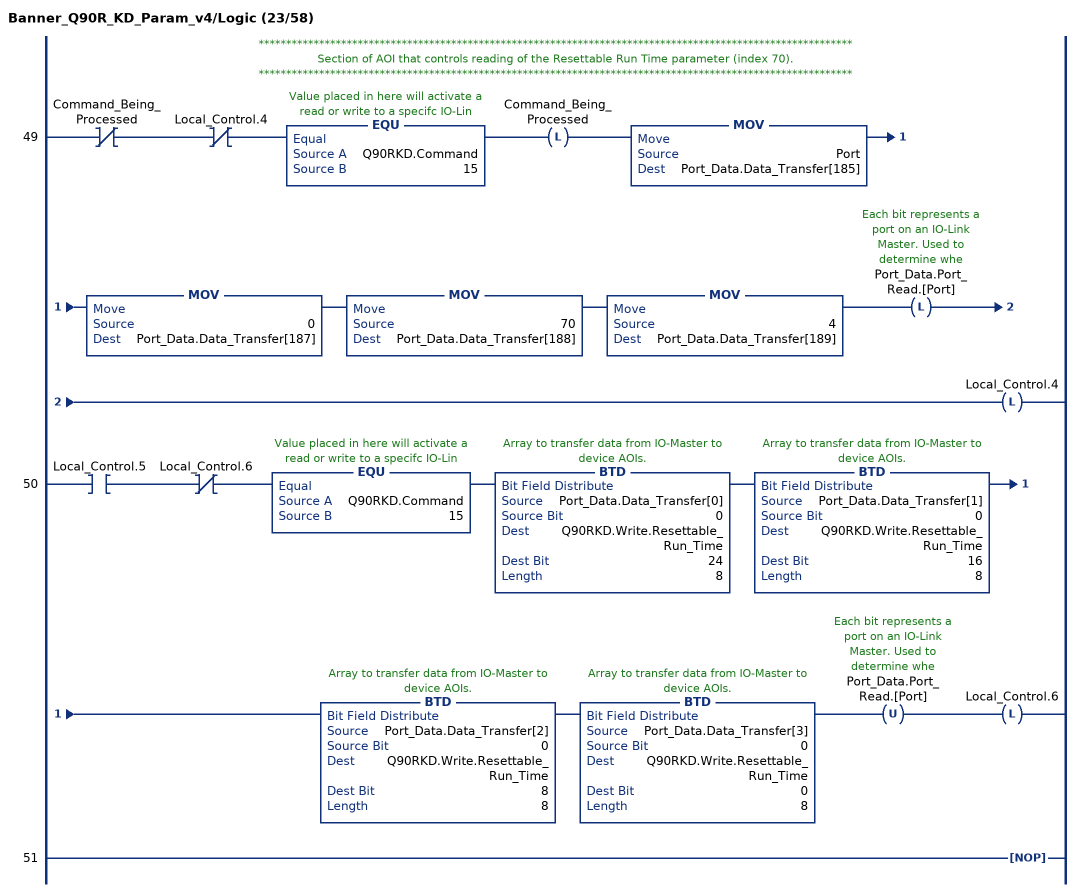
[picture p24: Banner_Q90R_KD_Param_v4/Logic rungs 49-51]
   // ************************************************************************************************************
   // Section of AOI that controls reading of the Resettable Run Time parameter (index 70).
   // ************************************************************************************************************
   49: XIO(Command_Being_Processed)XIO(Local_Control.4)EQU(Q90RKD.Command,15)OTL(Command_Being_Processed)MOV(Port,Port_Data.Data_Transfer[185])MOV(0,Port_Data.Data_Transfer[187])MOV(70,Port_Data.Data_Transfer[188])MOV(4,Port_Data.Data_Transfer[189])OTL(Port_Data.Port_Read.[Port])OTL(Local_Control.4);
   50: XIC(Local_Control.5)XIO(Local_Control.6)EQU(Q90RKD.Command,15)BTD(Port_Data.Data_Transfer[0],0,Q90RKD.Write.Resettable_Run_Time,24,8)BTD(Port_Data.Data_Transfer[1],0,Q90RKD.Write.Resettable_Run_Time,16,8)BTD(Port_Data.Data_Transfer[2],0,Q90RKD.Write.Resettable_Run_Time,8,8)BTD(Port_Data.Data_Transfer[3],0,Q90RKD.Write.Resettable_Run_Time,0,8)OTU(Port_Data.Port_Read.[Port])OTL(Local_Control.6);
   51: NOP();
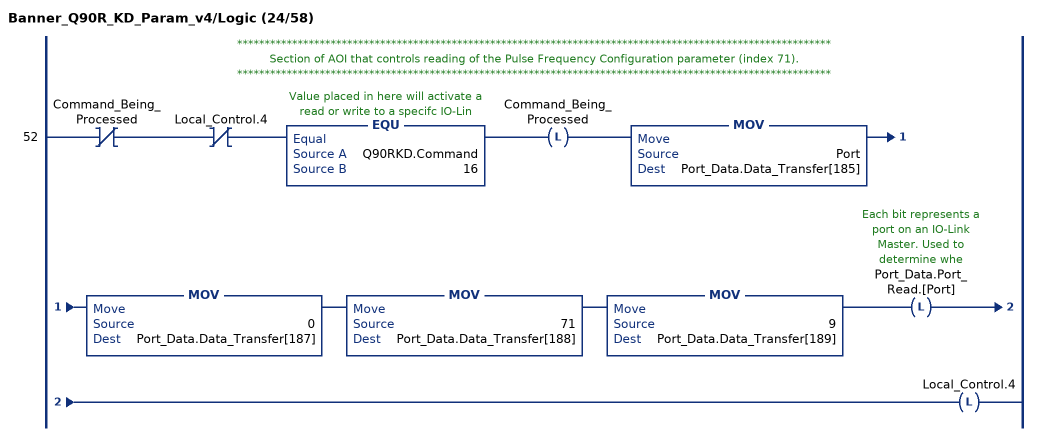
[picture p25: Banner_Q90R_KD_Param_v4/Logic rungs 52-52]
   // ************************************************************************************************************
   // Section of AOI that controls reading of the Pulse Frequency Configuration parameter (index 71).
   // ************************************************************************************************************
   52: XIO(Command_Being_Processed)XIO(Local_Control.4)EQU(Q90RKD.Command,16)OTL(Command_Being_Processed)MOV(Port,Port_Data.Data_Transfer[185])MOV(0,Port_Data.Data_Transfer[187])MOV(71,Port_Data.Data_Transfer[188])MOV(9,Port_Data.Data_Transfer[189])OTL(Port_Data.Port_Read.[Port])OTL(Local_Control.4);
